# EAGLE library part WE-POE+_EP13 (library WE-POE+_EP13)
Transformer for Power-over-Ethernet WE-PoE+ - Designed to meet 30W PoE+ objectives of IEEE802.3at - Frequency range: 250-400 kHz - Insulation voltage 1,5 kVAC/1 min - Input voltages 36V till 72V -- PoE+ Powered devices -- Ip phones -- WLAN-Access point -- Security cameras
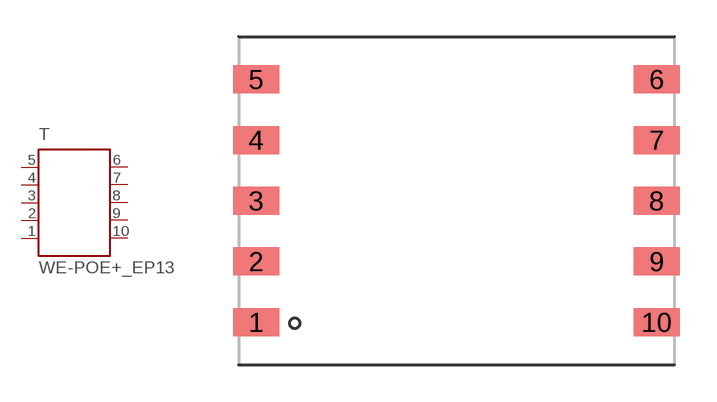
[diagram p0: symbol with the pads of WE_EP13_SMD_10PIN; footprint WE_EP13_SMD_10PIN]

Designator prefix T

## WE-POE+_EP13, WE-POE+_EP13-750310742 (MPN: 750310742; OC_FARNELL: 1849028; OC_NEWARK: 13T9828; PACKAGE: EP13; SUPPLIER: Wuerth Elektronik), WE-POE+_EP13-750310743 (MPN: 750310743; OC_FARNELL: 1849026; OC_NEWARK: 13T9829; PACKAGE: EP13; SUPPLIER: Wuerth Elektronik), WE-POE+_EP13-750310744 (MPN: 750310744; OC_FARNELL: 1849027; OC_NEWARK: 13T9830; PACKAGE: EP13; SUPPLIER: Wuerth Elektronik)  [WE_EP13_SMD_10PIN]
1  5  pas
2  4  pas
3  3  pas
4  2  pas
5  1  pas
6  10  pas
7  9  pas
8  8  pas
9  7  pas
10  6  pas

## Footprint WE_EP13_SMD_10PIN (pad centres in mm)
Transformer, EP13 SMD 10 Pin
smd 1.88 x 1.143: 1 -8.18,-4.96; 2 -8.18,-2.48; 3 -8.18,0; 4 -8.18,2.48; 5 -8.18,4.96; 6 8.18,4.96; 7 8.18,2.48; 8 8.18,0; 9 8.18,-2.48; 10 8.18,-4.96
